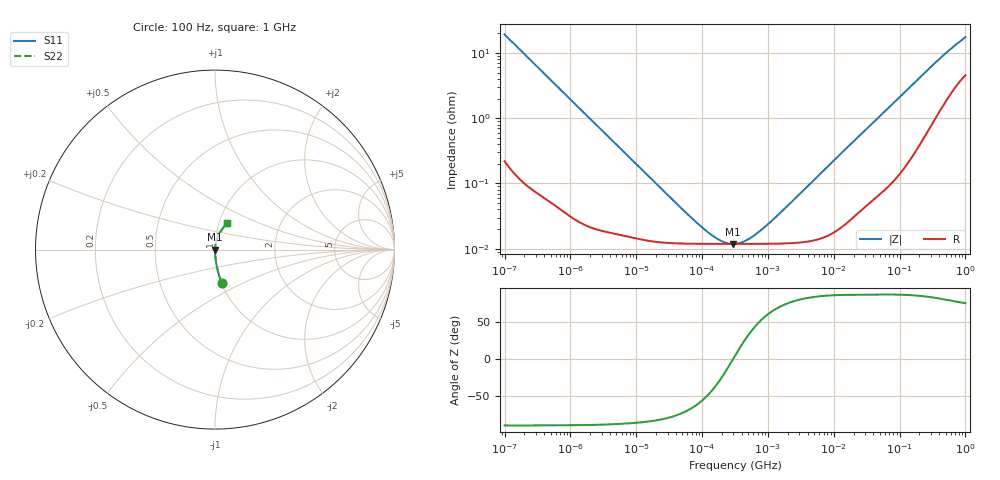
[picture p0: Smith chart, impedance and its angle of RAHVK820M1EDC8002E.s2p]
! RAHVK820M1EDC8002E  S-PARAMETER MODEL  (AEC-Q200 qualified)
! Model Generated by ELNA Corporation (http://www.ty-top.com)
! Version 1.0
! ELNA Control No.201026
! Copyright (c) 2020 ELNA CO.,LTD. All Rights Reserved.
! Products Name : CONDUCTIVE POLYMER HYBRID ALUMINUM ELECTROLYTIC CAPACITORS
! Characteristics :
!  Capacitance  :  82uF  ,  Rated voltage  :  16V
!  Operating Temp. Range  :  -55 to +125 degC  ,  Endurance  :  4000hr at 125 degC
!  Dimension D  :  6.3mm  ,  Dimension L  :  5.8mm
! Frequency Range : 100Hz - 1GHz
! External Node Assignments :
!  1  o---| |---o  2
# MHz S RI R 50
!Freq[MHz].  S11 Real  S11 Imag  S21 Real  S21 Imag  S12 Real  S12 Imag  S22 Real  S22 Imag
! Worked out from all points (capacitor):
!   401 points, 100 Hz to 1 GHz, reference 50 ohm
!   read as one part in series: C = 83.1 uF near 108 Hz
!   lowest |Z| = 11.9 mohm at 291.7 kHz (marker M1)
!   series resonance near 296.9 kHz, so ESL is about 3.5 nH
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0.0001  0.0373 -0.1839  0.9627 0.1839  0.9627 0.1839  0.0373 -0.1839
0.000113  0.0297 -0.1643  0.9703 0.1643  0.9703 0.1643  0.0297 -0.1643
0.000183  0.0119 -0.1033  0.9881 0.1033  0.9881 0.1033  0.0119 -0.1033
0.000309  0.00455 -0.0618  0.9954 0.0618  0.9954 0.0618  0.00455 -0.0618
0.001488  0.000414 -0.013  0.9996 0.013  0.9996 0.013  0.000414 -0.013
0.022131  0.000127 -0.000891  0.9999 0.000891  0.9999 0.000891  0.000127 -0.000891
0.068391  0.00012 -0.000275  0.9999 0.000275  0.9999 0.000275  0.00012 -0.000275
0.12517  0.000119 -0.000131  0.9999 0.000131  0.9999 0.000131  0.000119 -0.000131
0.194984  0.000119 -5.8e-05  0.9999 5.8e-05  0.9999 5.8e-05  0.000119 -5.8e-05
0.238506  0.000119 -2.96e-05  0.9999 2.96e-05  0.9999 2.96e-05  0.000119 -2.96e-05
0.291743  0.000119 -2.34e-06  0.9999 2.34e-06  0.9999 2.34e-06  0.000119 -2.34e-06
0.316228  0.000119 8.47e-06  0.9999 -8.47e-06  0.9999 -8.47e-06  0.000119 8.47e-06
0.386812  0.000119 3.59e-05  0.9999 -3.59e-05  0.9999 -3.59e-05  0.000119 3.59e-05
0.473151  0.000119 6.47e-05  0.9999 -6.47e-05  0.9999 -6.47e-05  0.000119 6.47e-05
0.737055  0.000119 0.000139  0.9999 -0.000139  0.9999 -0.000139  0.000119 0.000139
1.40443  0.00012 0.000303  0.9999 -0.000303  0.9999 -0.000303  0.00012 0.000303
4.704354  0.000134 0.00106  0.9999 -0.00106  0.9999 -0.00106  0.000134 0.00106
69.9842  0.00115 0.0148  0.9989 -0.0148  0.9989 -0.0148  0.00115 0.0148
176.8072  0.00446 0.0364  0.9955 -0.0364  0.9955 -0.0364  0.00446 0.0364
395.8221  0.018 0.0763  0.982 -0.0763  0.982 -0.0763  0.018 0.0763
668.3439  0.0407 0.1149  0.9593 -0.1149  0.9593 -0.1149  0.0407 0.1149
1000  0.0675 0.1494  0.9325 -0.1494  0.9325 -0.1494  0.0675 0.1494
